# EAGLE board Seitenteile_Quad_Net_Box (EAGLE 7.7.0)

Size 65 x 80 mm. Coordinates in mm from the lower left corner, seen from the top.
Outline: 90 segments
Copper layers (1*16): Top 0.035mm / dielectric 1.5mm / Bottom 0.035mm
Design rules "default": minimum track width 10mil, minimum drill 24mil, track to track 8mil, track to pad 8mil, pad to pad 8mil, via to via 8mil, smd to smd 8mil, copper to edge 40mil, drill to drill 8mil, minimum pad ring 10mil, minimum via ring 8mil, stop-mask expansion 4mil, vias tented up to drill 0mil, thermal gap 10mil

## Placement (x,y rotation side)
